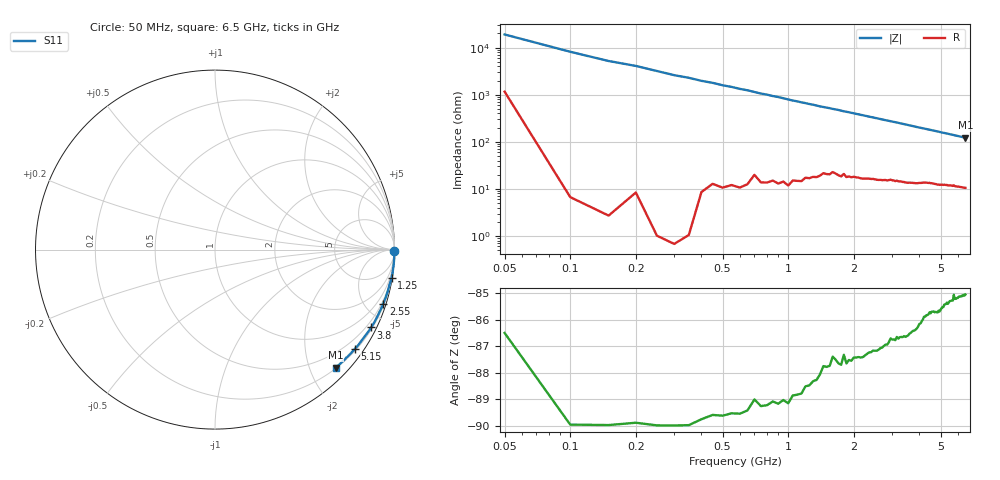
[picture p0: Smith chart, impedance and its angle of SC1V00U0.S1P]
! Infineon Technologies  Discrete & RF Semiconductors
! BAR63-02L
! Si PIN Diode in TSLP-2
! VR = 1 V
! S-Parameters:  March  2002
# GHz  S  MA  R  50
!  f  S11
! GHz  MAG  ANG
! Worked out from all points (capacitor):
!   130 points, 50 MHz to 6.5 GHz, reference 50 ohm
!   read as one part to ground: C = 194 fF near 50 MHz
!   lowest |Z| = 122 ohm at 6.5 GHz (marker M1)
!   S11 on the Smith chart (normalised r, x): 50 MHz: open; 1.25 GHz: 0, -13; 2.55 GHz: 0.31, -6.33; 3.8 GHz: 0.27, -4.23; 5.15 GHz: 0.24, -3.11; 6.5 GHz: 0.21, -2.43
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0.05  0.9997 -0.3
0.15  1 -1.1
0.35  1 -2.5
0.65  0.9992 -4.6
0.75  0.9988 -5.4
0.9  0.9984 -6.4
1.05  0.9974 -7.6
1.25  0.9959 -9.0
1.4  0.9941 -10.1
1.6  0.991 -11.4
1.7  0.9915 -12.0
1.8  0.9897 -12.8
1.85  0.9907 -13.1
2.2  0.988 -15.5
2.5  0.9852 -17.6
2.55  0.9849 -17.9
2.7  0.9834 -19.0
3.3  0.9774 -23.0
3.55  0.9754 -24.8
3.8  0.9724 -26.5
4.1  0.9676 -28.6
4.9  0.9587 -33.8
4.95  0.9586 -34.2
5.15  0.9556 -35.5
5.7  0.9492 -39.1
5.75  0.9466 -39.5
5.9  0.9472 -40.4
6.5  0.9413 -44.4
